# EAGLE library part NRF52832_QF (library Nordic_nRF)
nRF52832 Features Single chip, highly flexible, 2.4 GHz multi-protocol SoC 32-bit ARM Cortex-M4F Processor 1.7v to 3.6v operation 512kB flash + 64kB RAM Supports concurrent Bluetooth Smart/ANT protocol operation On-chip NFC tag for Out-of-Band (OOB) pairing Up to +4dBm output power -96dBm sensitivity, Bluetooth Smart Thread safe and run-time protected Event driven API On air compatible with nRF24L and nRF24AP series 2 data rates (2Mbps/1Mbps) PPI - maximum flexibility for power-efficient applications and code simplification Automated power management system with automatic power management of each peripheral Configurable I/O mapping for analog and digital I/O 3 x Master/Slave SPI 2 x Two-wire interface (I²C) UART (RTS/CTS) 3 x PWM AES HW encryption Real Time Counter (RTC) Digital microphone interface (PDM) On-chip balun Applications Internet of Things (IoT) Wearables SmartHome sensors Connected white goods Computer peripherals Voice-command smart remotes A4WP ‘Rezence’ wireless charging Beacons Sports and fitness sensors and hubs Connected health products Smart watches RC Toys Interactive games Building automation and sensor networks
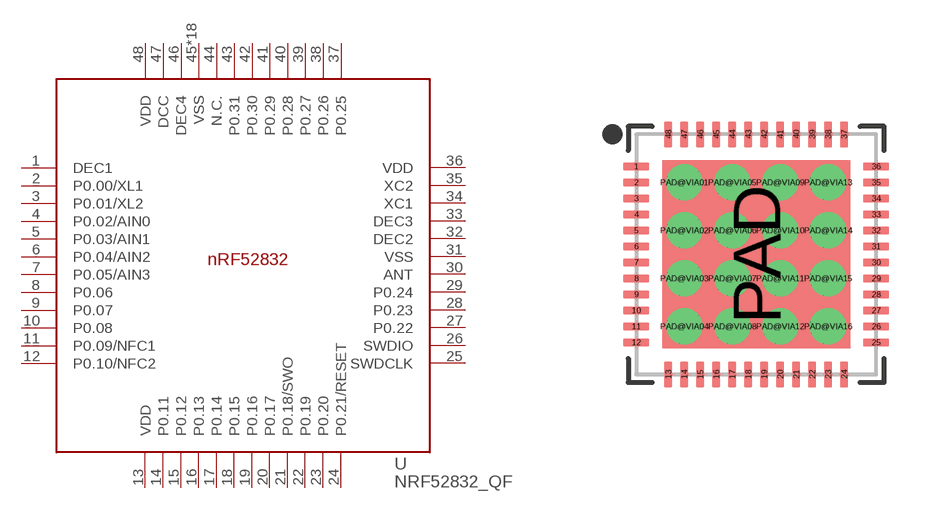
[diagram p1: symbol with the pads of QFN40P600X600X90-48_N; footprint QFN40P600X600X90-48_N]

Designator prefix -

## NRF52832_QF  [QFN40P600X600X90-48_N]
1  DEC1  pwr
2  P0.00/XL1
3  P0.01/XL2
4  P0.02/AIN0
5  P0.03/AIN1
6  P0.04/AIN2
7  P0.05/AIN3
8  P0.06
9  P0.07
10  P0.08
11  P0.09/NFC1
12  P0.10/NFC2
13  VDD  pwr
14  P0.11
15  P0.12
16  P0.13
17  P0.14
18  P0.15
19  P0.16
20  P0.17
21  P0.18/SWO
22  P0.19
23  P0.20
24  P0.21/RESET
25  SWDCLK  in
26  SWDIO
27  P0.22
28  P0.23
29  P0.24
30  ANT
31  VSS
32  DEC2
33  DEC3
34  XC1  in
35  XC2  out
36  VDD  pwr
37  P0.25
38  P0.26
39  P0.27
40  P0.28
41  P0.29
42  P0.30
43  P0.31
44  N.C.  nc
45  VSS  pwr
46  DEC4  pwr
47  DCC  out
48  VDD  pwr
PAD  VSS  pwr
PAD@VIA01  VSS  pwr
PAD@VIA02  VSS  pwr
PAD@VIA03  VSS  pwr
PAD@VIA04  VSS  pwr
PAD@VIA05  VSS  pwr
PAD@VIA06  VSS  pwr
PAD@VIA07  VSS  pwr
PAD@VIA08  VSS  pwr
PAD@VIA09  VSS  pwr
PAD@VIA10  VSS  pwr
PAD@VIA11  VSS  pwr
PAD@VIA12  VSS  pwr
PAD@VIA13  VSS  pwr
PAD@VIA14  VSS  pwr
PAD@VIA15  VSS  pwr
PAD@VIA16  VSS  pwr

## Footprint QFN40P600X600X90-48_N (pad centres in mm)
QFN40P600X600X90-48N QFN, 48-Leads Body 6.0x6.0mm (max) Pitch 0.40mm IPC Medium Density
smd 0.65 x 0.2: 1 -3,2.2; 2 -3,1.8; 3 -3,1.4; 4 -3,1; 5 -3,0.6; 6 -3,0.2; 7 -3,-0.2; 8 -3,-0.6; 9 -3,-1; 10 -3,-1.4; 11 -3,-1.8; 12 -3,-2.2; 25 3,-2.2; 26 3,-1.8; 27 3,-1.4; 28 3,-1; 29 3,-0.6; 30 3,-0.2; 31 3,0.2; 32 3,0.6; 33 3,1; 34 3,1.4; 35 3,1.8; 36 3,2.2
smd 0.2 x 0.65: 13 -2.2,-3; 14 -1.8,-3; 15 -1.4,-3; 16 -1,-3; 17 -0.6,-3; 18 -0.2,-3; 19 0.2,-3; 20 0.6,-3; 21 1,-3; 22 1.4,-3; 23 1.8,-3; 24 2.2,-3; 37 2.2,3; 38 1.8,3; 39 1.4,3; 40 1,3; 41 0.6,3; 42 0.2,3; 43 -0.2,3; 44 -0.6,3; 45 -1,3; 46 -1.4,3; 47 -1.8,3; 48 -2.2,3
smd 4.7 x 4.7: PAD 0,0
drill 0.4: PAD@VIA01 -1.8,1.8; PAD@VIA02 -1.8,0.6; PAD@VIA03 -1.8,-0.6; PAD@VIA04 -1.8,-1.8; PAD@VIA05 -0.6,1.8; PAD@VIA06 -0.6,0.6; PAD@VIA07 -0.6,-0.6; PAD@VIA08 -0.6,-1.8; PAD@VIA09 0.6,1.8; PAD@VIA10 0.6,0.6; PAD@VIA11 0.6,-0.6; PAD@VIA12 0.6,-1.8; PAD@VIA13 1.8,1.8; PAD@VIA14 1.8,0.6; PAD@VIA15 1.8,-0.6; PAD@VIA16 1.8,-1.8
